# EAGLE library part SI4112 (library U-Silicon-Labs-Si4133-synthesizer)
RF Synthesizer w/ integrated VCOs (IF OUT)
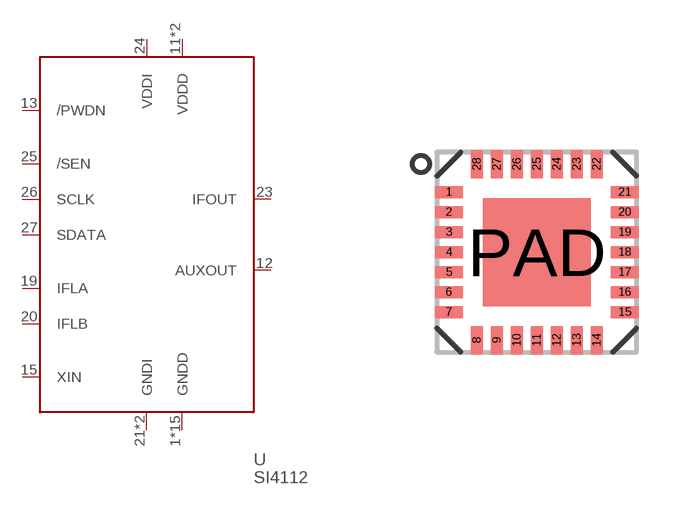
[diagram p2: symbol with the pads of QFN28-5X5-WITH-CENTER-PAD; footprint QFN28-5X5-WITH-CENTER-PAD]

Designator prefix U

## SI4112  [QFN28-5X5-WITH-CENTER-PAD]
1  GNDD  pwr
2  GNDD  pwr
3  GNDD  pwr
4  GNDD  pwr
5  GNDD  pwr
6  GNDD  pwr
7  GNDD  pwr
8  GNDD  pwr
9  GNDD  pwr
10  GNDD  pwr
11  VDDD  pwr
12  AUXOUT  out
13  /PWDN  in
14  GNDD  pwr
15  XIN  in
16  GNDD  pwr
17  VDDD  pwr
18  GNDD  pwr
19  IFLA  in
20  IFLB  in
21  GNDI  pwr
22  GNDI  pwr
23  IFOUT  out
24  VDDI  pwr
25  /SEN  in
26  SCLK  in
27  SDATA  in
28  GNDD  pwr
PAD  GNDD  pwr

## Footprint QFN28-5X5-WITH-CENTER-PAD (pad centres in mm)
smd 0.7 x 0.3: 1 -2.2,1.5; 2 -2.2,1; 3 -2.2,0.5; 4 -2.2,0; 5 -2.2,-0.5; 6 -2.2,-1; 7 -2.2,-1.5; 15 2.2,-1.5; 16 2.2,-1; 17 2.2,-0.5; 18 2.2,0; 19 2.2,0.5; 20 2.2,1; 21 2.2,1.5
smd 0.3 x 0.7: 8 -1.5,-2.2; 9 -1,-2.2; 10 -0.5,-2.2; 11 0,-2.2; 12 0.5,-2.2; 13 1,-2.2; 14 1.5,-2.2; 22 1.5,2.2; 23 1,2.2; 24 0.5,2.2; 25 0,2.2; 26 -0.5,2.2; 27 -1,2.2; 28 -1.5,2.2
smd 2.7 x 2.7: PAD 0,0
